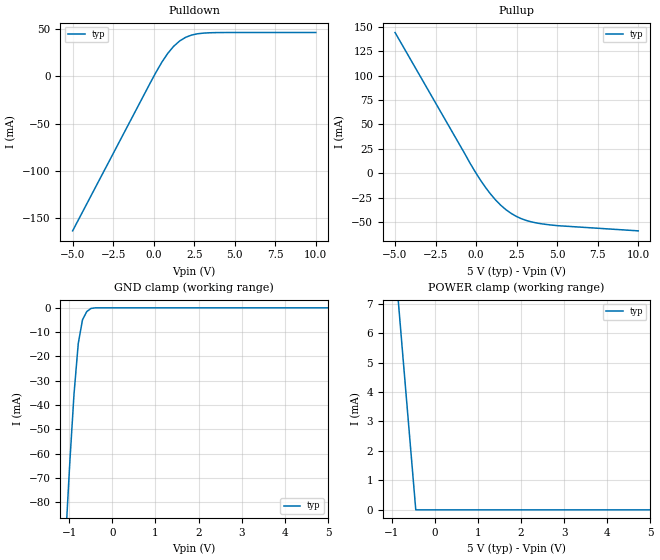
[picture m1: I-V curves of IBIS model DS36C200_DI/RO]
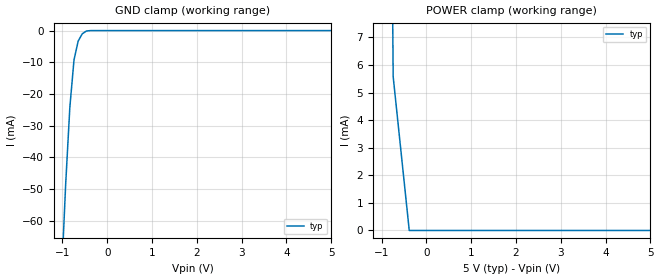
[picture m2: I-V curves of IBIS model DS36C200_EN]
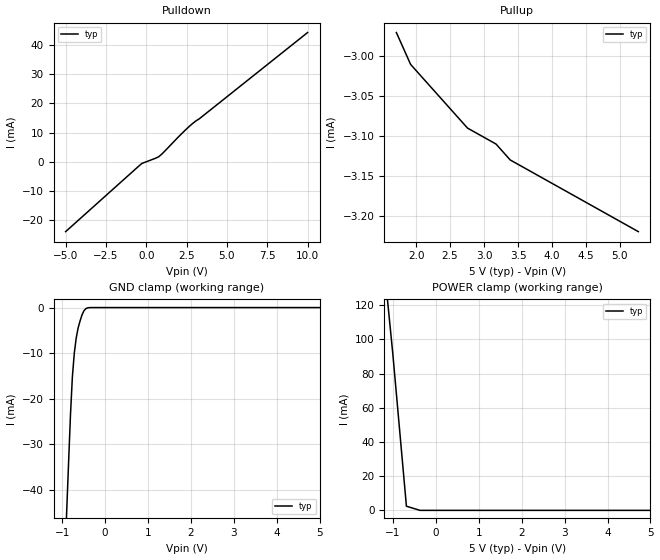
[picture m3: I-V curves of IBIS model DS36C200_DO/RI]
|   National Semiconductor Corporation
|   Interface Products Group
|   IBIS Model of DS36C200M
|   14L SOIC Package
[IBIS Ver]   2.1
[File name]   ds36c200.ibs
[Date]   5/27/98
[File Rev]   2.1
[Source]   Model Originated at National Semiconductor.
[Notes]   File created by MRW from emphirical data.
   File verified by SBH.
[Disclaimer]
(C) Copyright National Semiconductor Corporation 1994
   All rights reserved
   National Semiconductor Corporation hereby grants
the user of this IBIS model a non-exclusive, nontransferable
license to use this IBIS model under the following terms.
Before using this IBIS model, the user should read this
license.  If the user does not accept these terms,  the
IBIS model should be returned to National within 30 days.
   The user is granted this license only to use the
IBIS model and is not granted rights to sell, load, rent,
lease or license the IBIS model in whole or in part, or in
modified form to anyone other than user. User may modify
the IBIS model to suit its specific applications but rights
to derivative works and such modifications shall belong to
National.
   This IBIS model is provided on an "AS IS" basis and
National makes absolutely no warranty with respect to the
information contained herein.NATIONAL DISCLAIMS AND CUSTOMER
WAIVES ALL WARRANTIES, EXPRESS OR IMPLIED, INCLUDING
WARRANTIES OF MERCHANTABILITY OR FITNESS FOR A PARTICULAR
PURPOSE. The entire risk as to quality and performance is
with the Customer. ACCORDINGLY, IN NO EVENT SHALL THE
COMPANY BE LIABLE FOR ANY DAMAGES, WHETHER IN CONTRACT OR
TORT,INCLUDING ANY LOST PROFITS OR OTHER INCIDENTAL,
CONSEQUENTIAL, EXEMPLARY, OR PUNITIVE DAMAGES ARISING OUT
OF THE USE OR APPLICATION OF THE IBIS model provided in
this package.Further, National reserves the right to make
changes without notice to any product herein to improve
reliability, function, or design. National does not convey
any license under patent rights or any other intellectual
property rights, including those of third parties.
   National is not obligated to provide maintenance or support
for the licensed IBIS model.
Contact National at ATTN:INTERFACE APPLICATIONS/IBIS MODELS.
2900 Semiconductor Drive, M/S A2595, Santa Clara, CA 95052-8090
|   COMPONENT: DS36C200M
[Component]   DS36C200M
[Manufacturer]  National Semiconductor Corporation
[Package]
| variable   typ   min   max
R_pkg   50m   25m   75m
L_pkg   1.47n   1.05n   2.11n
C_pkg   0.28p   0.17p   0.40p
[Pin]   signal_name   model_name   R_pin   L_pin   C_pin
  1   DI/RO1   DS36C200_DI/RO   50m   1.47n   .28p
  2   Vcc   POWER   50m   1.47n   .28p
  3   DE   DS36C200_EN   50m   1.47n   .28p
  4   RE*   DS36C200_EN   50m   1.47n   .28p
  5   GND   GND   50m   1.47n   .28p
  6   NC   NC   50m   1.47n   .28p
  7   DI/RO2   DS36C200_DI/RO   50m   1.47n   .28p
  8   NC   NC   50m   1.47n   .28p
  9   NC   NC   50m   1.47n   .28p
  10   DO/RI2+   DS36C200_DO/RI   50m   1.47n   .28p
  11   DO/RI2-   DS36C200_DO/RI   50m   1.47n   .28p
  12   DO/RI1-   DS36C200_DO/RI   50m   1.47n   .28p
  13   DO/RI1+   DS36C200_DO/RI   50m   1.47n   .28p
  14   NC   NC   50m   1.47n   .28p
[Diff_pin]   inv_pin   vdiff   tdelay_typ   tdelay_min   tdelay_max
| The '+' pin is Diff_pin and the '-' pin is the inv_pin
10   11   NA   0 0 0
13   12   NA   0 0 0
| Models and submodels in the file (3): DS36C200_DI/RO (I/O), DS36C200_EN (Input), DS36C200_DO/RI (I/O)
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|   Driver Input/ Receiver Output MODEL {START}
[Model]   DS36C200_DI/RO
Model_type   I/O
|Signals   DI/RO1+,DI/RO1-,DI/RO2+,DI/RO2-
Vmeas = 1.5V   |Reference voltage for timing measurements
Cref = 8pF   |Timing specification test load capacitance value
Vref = 0   |Timing specification test load voltage; GND
Vinh = 2.0
Vinl = 0.8
|   typ   min   max
C_comp   1.0pF   NA   NA
|   typ   min   max
[Temperature Range]   25.0   NA   NA
[Voltage range]   5.0V   4.5V   5.5V
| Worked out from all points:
|   slope of the pulldown table from 0 to 0.75 V, typ, clamps not added: 34.7 ohm
|   slope of the pullup table from 0 to 0.75 V, typ, clamps not added: 41.2 ohm
|   GND clamp passes 1 mA (typ) near -0.55 V on its own axis
[Pulldown]
|   Voltage   I(typ)   I(min)   I(max)
-5V       -164mA     NA         NA
138.9mV   4.304mA    NA         NA
505.3mV   15.18mA    NA         NA
871.6mV   24.57mA    NA         NA
1.238V    32.09mA    NA         NA
1.604V    37.7mA     NA         NA
1.971V    41.53mA    NA         NA
2.337V    43.93mA    NA         NA
3.069V    46mA       NA         NA
10V       46.65mA    NA         NA
[Pullup]
|   Voltage   I(typ)   I(min)   I(max)
| Note that the[Pullup]voltage table is referenced to Vcc
| and is calculated using Vtable=Vcc - Vmeasured.
-5V       144mA      NA         NA
-52.63mV  1.444mA    NA         NA
578.9mV   -14.38mA   NA         NA
894.7mV   -21.28mA   NA         NA
1.526V    -32.71mA   NA         NA
1.842V    -37.21mA   NA         NA
2.158V    -40.93mA   NA         NA
2.789V    -46.37mA   NA         NA
3.421V    -49.66mA   NA         NA
4.053V    -51.62mA   NA         NA
5V        -53.47mA   NA         NA
10V       -58.8mA    NA         NA
[Power_clamp]
| Note that the[POWER_clamp]voltage table is referenced to Vcc
| and is calculated using Vtable=Vcc - Vmeasured.
|   Voltage   I(typ)   I(min)   I(max)
-5V       80.3mA     NA         NA
-740mV    5.277mA    NA         NA
-437.9mV  140nA      NA         NA
5V        0A         NA         NA
[GND_clamp]
|   Voltage   I(typ)   I(min)   I(max)
-5V       -1.15A     NA         NA
-1.083V   -96.09mA   NA         NA
-984.2mV  -63.91mA   NA         NA
-885.8mV  -35.46mA   NA         NA
-787.4mV  -14.69mA   NA         NA
-688.9mV  -4.911mA   NA         NA
-590.5mV  -1.549mA   NA         NA
-492.1mV  -255.1uA   NA         NA
-393.7mV  0A         NA         NA
5V        0A         NA         NA
[Ramp]
|   typ   min   max
dV/dt_r   4/1.5ns   NA   NA
dV/dt_f   4/1.5ns   NA   NA
R_load = 1MOhm   | note Represents an open
|   Driver Input/ Receiver Output MODEL {END}
|   Driver and Receiver Enable  MODEL {START}
[Model]   DS36C200_EN
Model_type   Input
|Signals   RE* and DE
Vinh = 2.0
Vinl = 0.8
|   typ   min   max
C_comp   1.0pF   NA   NA
|   typ   min   max
[Temperature Range]   25.0   NA   NA
[Voltage range]   5.0V   4.5V   5.5V
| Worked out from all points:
|   GND clamp passes 1 mA (typ) near -0.56 V on its own axis
[GND_clamp]
|   Voltage   I(typ)   I(min)   I(max)
-5V       -1.33A     NA         NA
-1.022V   -77.96mA   NA         NA
-928.9mV  -48.51mA   NA         NA
-836.1mV  -24.26mA   NA         NA
-743.2mV  -9.271mA   NA         NA
-650.3mV  -3.324mA   NA         NA
-557.4mV  -993.2uA   NA         NA
-464.5mV  -130.4uA   NA         NA
5V        0A         NA         NA
[Power_clamp]
| Note that the[POWER_clamp]voltage table is referenced to Vcc
| and is calculated using Vtable=Vcc - Vmeasured.
|   Voltage   I(typ)   I(min)   I(max)
-5V       846mA      NA         NA
-743.2mV  5.575mA    NA         NA
-384.2mV  98.6nA     NA         NA
5V        0A         NA         NA
|   Driver and Receiver Enable  MODEL {END}
|   Driver Output and Receiver Input  MODEL {START}
[Model]   DS36C200_DO/RI
Model_type   I/O
| Signals   DO/RI1+,DO/RI1-,DO/RI2+ and DO/RI2-
Vmeas = 1.2V   |Reference voltage for timing measurements
Cref = 5pF   |Timing specification test load capacitance value
Rref = 27.5
Vref = 1.2   |Timing specification test load voltage; GND
Vinh = 1.4
Vinl = 1.0
| variable   typ   min   max
C_comp   3.0pF   NA   NA
|   typ   min   max
[Temperature Range]   25.0   NA   NA
[Voltage range]   5.0V   4.5V   5.5V
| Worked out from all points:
|   slope of the pulldown table from 0 to 0.75 V, typ, clamps not added: 451 ohm
|   GND clamp passes 1 mA (typ) near -0.51 V on its own axis
[Pulldown]
|   Voltage   I(typ)   I(min)   I(max)
-5V       -24mA      NA         NA
-271.1mV  -600.5uA   NA         NA
776.3mV   1.705mA    NA         NA
2.871V    13.09mA    NA         NA
10V       44.3mA     NA         NA
[Pullup]
|   Voltage   I(typ)   I(min)   I(max)
| Note that the[Pullup]voltage table is referenced to Vcc
| and is calculated using Vtable=Vcc - Vmeasured.
|   10.00V   -0.00322   NA   NA
1.71V     -2.97mA    NA         NA
1.919V    -3.01mA    NA         NA
2.757V    -3.09mA    NA         NA
3.176V    -3.11mA    NA         NA
3.386V    -3.13mA    NA         NA
5.271V    -3.22mA    NA         NA
|   -5.00V   -0.00297   NA   NA
[GND_clamp]
|   Voltage   I(typ)   I(min)   I(max)
| Outputs in Tri-state.
-5V       -1.04A     NA         NA
-850mV    -34.26mA   NA         NA
-805.3mV  -23.58mA   NA         NA
-760.5mV  -15.17mA   NA         NA
-715.8mV  -9.968mA   NA         NA
-671.1mV  -6.649mA   NA         NA
-626.3mV  -4.453mA   NA         NA
-536.8mV  -1.614mA   NA         NA
-492.1mV  -717.3uA   NA         NA
-447.4mV  -235.6uA   NA         NA
-313.2mV  0A         NA         NA
5V        0A         NA         NA
[POWER_clamp]
|   Voltage   I(typ)   I(min)   I(max)
| Note that the[POWER_clamp]voltage table is referenced to Vcc
| and is calculated using Vtable=Vcc - Vmeasured.
| Outputs in Tri-state.
-5V       1.11A      NA         NA
-1V       91.29mA    NA         NA
-684.2mV  2.428mA    NA         NA
-368.4mV  26.9nA     NA         NA
-52.63mV  0A         NA         NA
263.2mV   0A         NA         NA
5V        0A         NA         NA
[Ramp]
| Note: Ramp rate measured on single-ended Driver Output.
|   typ   min   max
dV/dt_r   0.21/400p   NA   NA
dV/dt_f   0.21/389p   NA   NA
R_load = 55Ohm | Note: This 55 Ohm is across the two driver output
